(* Logix 5000 AddOnInstructionDefinition export EH_Cerabar_PMP23_IOL; software revision 38.00 *)

TYPE EH_CommAOI_Data :
STRUCT
   Device_Comm_Error : BOOL;
   CommSuccess : BOOL;
   CommFailed : BOOL;
   CommTimeOut : BOOL;
   StateDone : BOOL;
   NewState : BOOL;
   OldState : SINT;
   PortSize : SINT;
   DevicePort : SINT;
   MaxState : SINT;
   State : SINT;
   VendorID : INT;
   DeviceID : DINT;
   CyclicData : INT[16];
   AcyclicData : DINT[8];
   ReplayIndex : INT;
   AOI_Diagnostic : DINT;
   ConnectionStatus : DINT;
   OutputData : INT[16];
END_STRUCT
END_TYPE

ADD_ON_INSTRUCTION EH_Cerabar_PMP23_IOL   (* revision 1.0, vendor Endress+Hauser *)
// Cerabar PMP23 Rev 1 IO-Link
// Cerabar PMP23 Rev 2 IO-Link
// Cerabar PMP23 Rev 3 IO-Link
VAR_IN_OUT
   DataToSend : INT[10]; {required}
   CommAOIBusy : DINT; {required}
   ActiveComPort : DINT; {required}
   DeviceAOISendRequest : DINT; {required}
   CommError : INT; {required}
   DeviceData : EH_CommAOI_Data; {required}
END_VAR
VAR_INPUT
   iExecuteRisingEdge : BOOL; {visible}
   iGetZero : BOOL; {visible}
   iSetUnit : DINT; {visible}
END_VAR
VAR_OUTPUT
   qVendor_ID : DINT; {access Read Only, visible}
   qDevice_ID : DINT; {access Read Only, visible}
   qPressure : REAL; {visible}
   qCondensedStatus : USINT; {access Read Only, visible}
   qS_Out_1 : BOOL; {access Read Only, visible}
   qS_Out_2 : BOOL; {access Read Only, visible}
   qUnit : DINT; {access Read Only, visible}
   qAOI_Diagnostic : DINT; {access Read Only, visible}
END_VAR
VAR_IN_OUT
   qActual_Diagnostics_String : STRING; {required}
END_VAR
VAR_OUTPUT
   qActual_Diagnostics_Code : DINT; {access Read Only, visible}
END_VAR
VAR_IN_OUT
   qLast_Diagnostics_String : STRING; {required}
END_VAR
VAR_OUTPUT
   qLast_Diagnostics_Code : DINT; {access Read Only, visible}
   qCommunicationBusy : DINT; {visible}
   qCommError : DINT; {access Read Only, visible}
   qDeviceConnectionError : BOOL; {access None, visible}
END_VAR
VAR
   Calc_DID : DINT; {access None}
   Calc_VID : DINT; {access None}
   Calc_Data : DINT; {access None}
   Test : DINT; {access None}
   Pressure_DINT : DINT; {access None}
   Calc_Pressure : DINT; {access None}
   Calc_CondenStatus : DINT; {access None}
   CMD_Index : INT; {access None}
   CMD_Subindex : INT; {access None}
   CMD_ByteLength : INT; {access None}
   qDevice_ID_select : INT; {access None}
   Trigger : BOOL; {access None}
   CMD_Rd : BOOL; {access None}
   CMD_Wr : BOOL; {access None}
   Calc_Out : DINT; {access None}
   UnitSelection : REAL; {access None}
   InputByteLength : DINT;
   LocalChannel : BOOL; {access None}
   StateMin : DINT; {access None}
   StateMax : DINT; {access None}
   UseDeviceUnit : BOOL; {access None}
   ActiveAOI : BOOL; {access None}
   firstTimeDone : BOOL; {access None}
   AOI_Prio : BOOL; {access None}
   Calc_Connection_Status : DINT; {access None}
   DeviceID1 : DINT; {access None}
   DeviceID2 : DINT; {access None}
   DeviceID3 : DINT; {access None}
   qPressureTemp : REAL; {access None}
   FALSE : BOOL; {access None}
   TRUE : BOOL := 1; {access None}
END_VAR

ROUTINE Logic   (* structured text *)
// PMP23 Communication via AL1323
   // =======================================================================
   // Endress+Hauser Digital Solutions
   // ©Copyright (2024) All Rights Reserved
   // =======================================================================
   // Name:                EH_Cerabar_PMP23_IOL
   // Version:             1.0
   // Datum:               11.2025
   // Library:             01.01.00
   // Engineering:         Studio5000 V38.00.00
   // Author:              EH
   // =======================================================================
   
   
   qAOI_Diagnostic := DeviceData.AOI_Diagnostic;
   qCommunicationBusy := CommAOIBusy;
   DeviceID1 := 256;  //PMP 23 Rev 1
   DeviceID2 := 257;  //PMP 23 Rev 2
   DeviceID3 := 258;  //PMP 23 Rev 3
   StateMin := 0;
   DeviceData.MaxState := 6;
   
   if DeviceData.DevicePort = 0 or DeviceData.DeviceID < DeviceID1 or DeviceData.DeviceID > DeviceID3 or DeviceData.ConnectionStatus <> 1 then
   
   	qVendor_ID	:= 0;
   	qDevice_ID	:= 0;
   	qPressure	:= 0;
   	qS_Out_1	:= 0;
   	qS_Out_2	:= 0;
   	qCondensedStatus	:= 0;
   	qActual_Diagnostics_Code	:= 0;
   	qLast_Diagnostics_Code	:= 0;
   	qLast_Diagnostics_String	:= '';
   
   	if DeviceData.DevicePort = 0 then
   
   		qActual_Diagnostics_String	:= 'Device Port is Zero';
   		DeviceData.AOI_Diagnostic.1 := TRUE;
   
   	elsif DeviceData.ConnectionStatus <> 1 then
   
   		qActual_Diagnostics_String	:= 'No Device connected';
   		qDeviceConnectionError := TRUE;
   
   	elsif DeviceData.DeviceID < DeviceID1 or DeviceData.DeviceID > DeviceID3  then
   
   		qActual_Diagnostics_String	:= 'Wrong DeviceID';
   		DeviceData.AOI_Diagnostic.2 := TRUE;
   		qVendor_ID := DeviceData.VendorID;
   		qDevice_ID := DeviceData.DeviceID;
   
   	end_if;
   
   else
   
   	if qActual_Diagnostics_Code = 0 then
   
   		qActual_Diagnostics_String	:= '--------';
   
   	end_if;
   
   	if qLast_Diagnostics_Code = 0 then
   
   		qLast_Diagnostics_String	:= '--------';
   
   	end_if;
   
   	DeviceData.AOI_Diagnostic.1 := FALSE;
   	qDeviceConnectionError := FALSE;
   	DeviceData.AOI_Diagnostic.2  := FALSE;
   
   end_if;
   
   
   if not DeviceData.AOI_Diagnostic.0
   	and not qDeviceConnectionError
   	and not DeviceData.AOI_Diagnostic.2
   	and DeviceData.DevicePort > 0 or ActiveAOI and qDeviceConnectionError then
   
   	//*********************************
   	//Vendor ID
   	//*********************************
   
   	qVendor_ID := DeviceData.VendorID;
   
   	//*********************************
   	//Device ID
   	//*********************************
   
   	qDevice_ID := DeviceData.DeviceID;
   
   	if not UseDeviceUnit then
   
   		CASE iSetUnit OF
   
   			//*********************************
   			0: // Bar
   			//*********************************
   			UnitSelection := 10000.0;
   
   			//*********************************
   			1: // kPa
   			//*********************************
   			UnitSelection := 100.0;
   
   			//*********************************
   			2: // psi
   			//*********************************
   			UnitSelection := 1000.0;
   
   			//*********************************
   			3: // MPa
   			//*********************************
   			UnitSelection := 100000.0;
   
   		end_case;
   
   	end_if;
   
   	//*********************************
   	//Process Data Pressure
   	//*********************************
   	if DeviceData.DeviceID = DeviceID1 then
   
   		qDevice_ID_select := 1;
   
   	elsif DeviceData.DeviceID = DeviceID2 then
   
   		qDevice_ID_select := 2;
   
   	elsif DeviceData.DeviceID = DeviceID3 then
   
   		qDevice_ID_select := 3;
   
   	else
   
   		qDevice_ID_select := 0;
   
   	end_if;
   
   	case qDevice_ID_select of  // check for Different Version
   
   		//*********************************
   	    1: // PMP 23 Rev 1
   	    //*********************************
   
   		Calc_Pressure 	:= 0+((DeviceData.DevicePort-1)*InputByteLength);  // Value  95 + Protnumber x Datalength in Byte
   
   		Pressure_DINT :=  DeviceData.CyclicData[Calc_Pressure+1];
   		Pressure_DINT.8 :=  DeviceData.CyclicData[Calc_Pressure+1].8;
   		Pressure_DINT.9 :=  DeviceData.CyclicData[Calc_Pressure+1].9;
   		Pressure_DINT.10 :=  DeviceData.CyclicData[Calc_Pressure+1].10;
   		Pressure_DINT.11 :=  DeviceData.CyclicData[Calc_Pressure+1].11;
   		Pressure_DINT.12 :=  DeviceData.CyclicData[Calc_Pressure+1].12;
   		Pressure_DINT.13 :=  DeviceData.CyclicData[Calc_Pressure+1].13;
   		Pressure_DINT.14 :=  DeviceData.CyclicData[Calc_Pressure+1].14;
   		Pressure_DINT.15 :=  DeviceData.CyclicData[Calc_Pressure+1].15;
   		Pressure_DINT.16 :=  DeviceData.CyclicData[Calc_Pressure].0;
   		Pressure_DINT.17 :=  DeviceData.CyclicData[Calc_Pressure].1;
   		Pressure_DINT.18 :=  DeviceData.CyclicData[Calc_Pressure].2;
   		Pressure_DINT.19 :=  DeviceData.CyclicData[Calc_Pressure].3;
   		Pressure_DINT.20 :=  DeviceData.CyclicData[Calc_Pressure].4;
   		Pressure_DINT.21 :=  DeviceData.CyclicData[Calc_Pressure].5;
   		Pressure_DINT.22 :=  DeviceData.CyclicData[Calc_Pressure].5;
   		Pressure_DINT.23 :=  DeviceData.CyclicData[Calc_Pressure].5;
   		Pressure_DINT.24 :=  DeviceData.CyclicData[Calc_Pressure].5;
   		Pressure_DINT.25 :=  DeviceData.CyclicData[Calc_Pressure].5;
   		Pressure_DINT.26 :=  DeviceData.CyclicData[Calc_Pressure].5;
   		Pressure_DINT.27 :=  DeviceData.CyclicData[Calc_Pressure].5;
   		Pressure_DINT.28 :=  DeviceData.CyclicData[Calc_Pressure].5;
   		Pressure_DINT.29 :=  DeviceData.CyclicData[Calc_Pressure].5;
   		Pressure_DINT.30 :=  DeviceData.CyclicData[Calc_Pressure].5;
   		Pressure_DINT.31 :=  DeviceData.CyclicData[Calc_Pressure].5;
   
   
   		qPressure := Pressure_DINT;
   		qPressure := qPressure / UnitSelection;
   
   		//*********************************
   	    2: // PMP 23 Rev 2
   	    //*********************************
   
   		Calc_Pressure 	:= 0+((DeviceData.DevicePort-1)*InputByteLength);
   
   		Pressure_DINT :=  DeviceData.CyclicData[Calc_Pressure+1];
   		Pressure_DINT.8 :=  DeviceData.CyclicData[Calc_Pressure+1].8;
   		Pressure_DINT.9 :=  DeviceData.CyclicData[Calc_Pressure+1].9;
   		Pressure_DINT.10 :=  DeviceData.CyclicData[Calc_Pressure+1].10;
   		Pressure_DINT.11 :=  DeviceData.CyclicData[Calc_Pressure+1].11;
   		Pressure_DINT.12 :=  DeviceData.CyclicData[Calc_Pressure+1].12;
   		Pressure_DINT.13 :=  DeviceData.CyclicData[Calc_Pressure+1].13;
   		Pressure_DINT.14 :=  DeviceData.CyclicData[Calc_Pressure+1].14;
   		Pressure_DINT.15 :=  DeviceData.CyclicData[Calc_Pressure+1].15;
   		Pressure_DINT.16 :=  DeviceData.CyclicData[Calc_Pressure].0;
   		Pressure_DINT.17 :=  DeviceData.CyclicData[Calc_Pressure].1;
   		Pressure_DINT.18 :=  DeviceData.CyclicData[Calc_Pressure].2;
   		Pressure_DINT.19 :=  DeviceData.CyclicData[Calc_Pressure].3;
   		Pressure_DINT.20 :=  DeviceData.CyclicData[Calc_Pressure].4;
   		Pressure_DINT.21 :=  DeviceData.CyclicData[Calc_Pressure].5;
   		Pressure_DINT.22 :=  DeviceData.CyclicData[Calc_Pressure].6;
   		Pressure_DINT.23 :=  DeviceData.CyclicData[Calc_Pressure].7;
   		Pressure_DINT.24 :=  DeviceData.CyclicData[Calc_Pressure].8;
   		Pressure_DINT.25 :=  DeviceData.CyclicData[Calc_Pressure].9;
   		Pressure_DINT.26 :=  DeviceData.CyclicData[Calc_Pressure].10;
   		Pressure_DINT.27 :=  DeviceData.CyclicData[Calc_Pressure].11;
   		Pressure_DINT.28 :=  DeviceData.CyclicData[Calc_Pressure].12;
   		Pressure_DINT.29 :=  DeviceData.CyclicData[Calc_Pressure].13;
   		Pressure_DINT.30 :=  DeviceData.CyclicData[Calc_Pressure].13;
   		Pressure_DINT.31 :=  DeviceData.CyclicData[Calc_Pressure].13;
   
   		qPressure := Pressure_DINT;
   		qPressure := qPressure / UnitSelection;
   
   		//*********************************
   	    3: // PMP23 Rev 3
   	    //*********************************
   
   		Calc_Pressure 	:= 0+((DeviceData.DevicePort-1)*InputByteLength);
   		Calc_CondenStatus := 2+((DeviceData.DevicePort-1)*InputByteLength);
   
   		Pressure_DINT :=  DeviceData.CyclicData[Calc_Pressure+1];
   		Pressure_DINT.8 :=  DeviceData.CyclicData[Calc_Pressure+1].8;
   		Pressure_DINT.9 :=  DeviceData.CyclicData[Calc_Pressure+1].9;
   		Pressure_DINT.10 :=  DeviceData.CyclicData[Calc_Pressure+1].10;
   		Pressure_DINT.11 :=  DeviceData.CyclicData[Calc_Pressure+1].11;
   		Pressure_DINT.12 :=  DeviceData.CyclicData[Calc_Pressure+1].12;
   		Pressure_DINT.13 :=  DeviceData.CyclicData[Calc_Pressure+1].13;
   		Pressure_DINT.14 :=  DeviceData.CyclicData[Calc_Pressure+1].14;
   		Pressure_DINT.15 :=  DeviceData.CyclicData[Calc_Pressure+1].15;
   		Pressure_DINT.16 :=  DeviceData.CyclicData[Calc_Pressure].0;
   		Pressure_DINT.17 :=  DeviceData.CyclicData[Calc_Pressure].1;
   		Pressure_DINT.18 :=  DeviceData.CyclicData[Calc_Pressure].2;
   		Pressure_DINT.19 :=  DeviceData.CyclicData[Calc_Pressure].3;
   		Pressure_DINT.20 :=  DeviceData.CyclicData[Calc_Pressure].4;
   		Pressure_DINT.21 :=  DeviceData.CyclicData[Calc_Pressure].5;
   		Pressure_DINT.22 :=  DeviceData.CyclicData[Calc_Pressure].6;
   		Pressure_DINT.23 :=  DeviceData.CyclicData[Calc_Pressure].7;
   		Pressure_DINT.24 :=  DeviceData.CyclicData[Calc_Pressure].8;
   		Pressure_DINT.25 :=  DeviceData.CyclicData[Calc_Pressure].9;
   		Pressure_DINT.26 :=  DeviceData.CyclicData[Calc_Pressure].10;
   		Pressure_DINT.27 :=  DeviceData.CyclicData[Calc_Pressure].11;
   		Pressure_DINT.28 :=  DeviceData.CyclicData[Calc_Pressure].12;
   		Pressure_DINT.29 :=  DeviceData.CyclicData[Calc_Pressure].13;
   		Pressure_DINT.30 :=  DeviceData.CyclicData[Calc_Pressure].14;
   		Pressure_DINT.31 :=  DeviceData.CyclicData[Calc_Pressure].15;
   
   		COP(Pressure_DINT,qPressureTemp,1);
   
   		case qUnit of
   
   			//*********************************
   			0: // bar
   			//*********************************
   			qPressure := qPressureTemp / 100000;
   
   			//*********************************
   			1: // kPa
   			//*********************************
   			qPressure := qPressureTemp / 1000;
   
   			//*********************************
   			2: // psi
   			//*********************************
   			qPressure := qPressureTemp / 6895;
   
   			//*********************************
   			3: // MPA
   			//*********************************
   			qPressure := qPressureTemp / 1000000;
   
   			else // Base unit, Pa
   				qPressure := qPressureTemp;
   
   		end_case;
   
   	end_case;
   
   	//*********************************
   	// Process Parameter State IO1
   	//*********************************
   
   	if qDevice_ID = DeviceID1 then
   
   		qS_Out_1 :=  DeviceData.CyclicData[Calc_Pressure].6;
   		qS_Out_2 := 0;  // not supported
   
   	elsif qDevice_ID = DeviceID2 then
   
   		qS_Out_1 :=  DeviceData.CyclicData[Calc_Pressure].14;
   		qS_Out_2 := 0; // not supported
   
   	elsif qDevice_ID = DeviceID3 then
   
   		qS_Out_1 :=  DeviceData.CyclicData[Calc_CondenStatus].0;
   		qS_Out_2 :=  DeviceData.CyclicData[Calc_CondenStatus].1;
   
   	end_if;
   
   	//*********************************
   	// Process Parameter State IO1
   	//*********************************
   
   		if qDevice_ID = DeviceID3 then
   
   			qCondensedStatus.0 := DeviceData.CyclicData[Calc_CondenStatus].8;
   			qCondensedStatus.1 := DeviceData.CyclicData[Calc_CondenStatus].9;
   			qCondensedStatus.2 := DeviceData.CyclicData[Calc_CondenStatus].10;
   			qCondensedStatus.3 := DeviceData.CyclicData[Calc_CondenStatus].11;
   			qCondensedStatus.4 := DeviceData.CyclicData[Calc_CondenStatus].12;
   			qCondensedStatus.5 := DeviceData.CyclicData[Calc_CondenStatus].13;
   			qCondensedStatus.6 := DeviceData.CyclicData[Calc_CondenStatus].14;
   			qCondensedStatus.7 := DeviceData.CyclicData[Calc_CondenStatus].15;
   
   		end_if;
   
   	//*********************************
   	// Checking for CommBlockBusy
   	//*********************************
   
   
   	if iExecuteRisingEdge and DeviceData.State = 0 then
   
   		DeviceAOISendRequest.[DeviceData.DevicePort] := 1;
   
   	end_if;
   
   
   	if ActiveComPort = DeviceData.DevicePort then
   
   		AOI_Prio :=1;
   	else
   
   		AOI_Prio := 0;
   	end_if;
   
   
   	if CommAOIBusy = 1 and iExecuteRisingEdge and DeviceData.State = 0 and AOI_Prio then
   
   		ActiveAOI := 1;
   
   
   	end_if;
   
   
   	qCommunicationBusy := CommAOIBusy;
   	qAOI_Diagnostic := DeviceData.AOI_Diagnostic;
   
   	if  ActiveAOI and qDeviceConnectionError then
   
   		DeviceData.State := DeviceData.MaxState;
   
   	end_if;
   
   	//*********************************
   	// State machine
   	//*********************************
   
   
   	if ActiveAOI or DeviceData.State = DeviceData.MaxState then
   
   		case DeviceData.State of
   
   		    //*********************************
   		    0: // Idle
   		    //*********************************
   
   			    // Initializing reset to O for CMD Relevant Settings
   			    Trigger := 0;
   				CMD_Index := 0;
   				CMD_Subindex := 0;
   				CMD_Wr := 0;
   				CMD_Rd := 0;
   			    CMD_ByteLength := 0;
   
   				if DeviceData.DevicePort = ActiveComPort then // check if Device is Active to reset success
   						DeviceData.CommSuccess := 0;
   						DeviceData.CommTimeOut := 0;
   						DeviceData.NewState := 1;
   						DeviceData.StateDone := 0;
   				end_if;
   
   			    // Wait for trigger
   			    if iExecuteRisingEdge and ActiveComPort = DeviceData.DevicePort then
   
   					DeviceData.AOI_Diagnostic := 0;
   					DeviceData.State := DeviceData.State + 1;
   
   			    end_if;
   
   			//*********************************
   			1: // Set Unit
   			//*********************************
   
   				CMD_Index := 67;
   				CMD_Subindex := 0;
   				CMD_Wr := 1;								// Only Read or Write can be active = 1
   				CMD_Rd := 0;
   				CMD_ByteLength := 1;
   				DataToSend[6]:= 0;
   				DataToSend[7]:= 0;
   
   		        if iSetUnit >= 0 AND iSetUnit < 4 then		// Check if the value from outside is usable if not error set an go to next Step
   
   				   DataToSend[6].0 := iSetUnit.0;
   				   DataToSend[6].1 := iSetUnit.1;
   				   DataToSend[6].2 := iSetUnit.2;
   				   DataToSend[6].3 := iSetUnit.3;
   				   Trigger := 1;
   
   				   if DeviceData.NewState then
   
   						DeviceData.StateDone := 1;
   
   					end_if;
   
   				else
   
   		            DeviceData.AOI_Diagnostic.[DeviceData.State+7] := 1;
   					DeviceData.OldState := DeviceData.State;
   			        DeviceData.State := DeviceData.State + 1;
   					DeviceData.CommSuccess := 0;
   					DeviceData.AcyclicData[0] := 0;
   					DeviceData.NewState := 1;
   
   			    end_if;
   
   				if  DeviceData.CommSuccess and DeviceData.ReplayIndex = CMD_Index then
   
   					Trigger := 0;
   					DeviceData.OldState := DeviceData.State;
   			        DeviceData.State := DeviceData.State + 1;
   					DeviceData.CommSuccess := 0;
   					DeviceData.AcyclicData[0] := 0;
   					DeviceData.NewState := 1;
   
   				 elsif DeviceData.CommTimeOut then
   
   					DeviceData.AOI_Diagnostic.[DeviceData.State+7] := 1;
   					DeviceData.OldState := DeviceData.State;
   			        DeviceData.State := DeviceData.State + 1;
   					DeviceData.CommTimeOut := 0;
   					DeviceData.AcyclicData[0] := 0;
   					DeviceData.NewState := 1;
   
   			    end_if;
   
   		    //*********************************
   		    2: // Get Zero
   		    //*********************************
   
   		        CMD_Index := 69;
   		        CMD_Subindex := 0;
   		        CMD_Wr := 1;
   				CMD_Rd := 0;
   		        CMD_ByteLength := 1;
   				DataToSend[6]:= 0;
   				DataToSend[7]:= 0;
   
   				if DeviceData.NewState then
   
   					DeviceData.StateDone := 1;
   
   				end_if;
   
   				if iGetZero then
   
   					DataToSend[6].0 := 1;
   				else
   
   					DataToSend[6].0 := 0;
   				end_if;
   
   				Trigger := 1;
   
   				if  DeviceData.CommSuccess and DeviceData.ReplayIndex = CMD_Index then
   
   					Trigger := 0;
   					DeviceData.OldState := DeviceData.State;
   			        DeviceData.State := DeviceData.State + 1;
   					DeviceData.CommSuccess := 0;
   					DeviceData.AcyclicData[0] := 0;
   					DeviceData.NewState := 1;
   
   				 elsif DeviceData.CommTimeOut then
   
   					DeviceData.AOI_Diagnostic.[DeviceData.State+7] := 1;
   					DeviceData.OldState := DeviceData.State;
   			        DeviceData.State := DeviceData.State + 1;
   					DeviceData.CommTimeOut := 0;
   					DeviceData.AcyclicData[0] := 0;
   					DeviceData.NewState := 1;
   
   			    end_if;
   
   			//*********************************
   		    3: // Read Unit Set from Device
   		    //*********************************
   
   				CMD_Index := 67;
   		        CMD_Subindex := 0;
   		        CMD_Wr := 0;
   				CMD_Rd := 1;
   		        CMD_ByteLength := 1;
   				DataToSend[6]:= 0;
   				DataToSend[7]:= 0;
   				Trigger := 1;
   
   				if DeviceData.NewState then
   
   					DeviceData.StateDone := 1;
   
   				end_if;
   
   				if  DeviceData.CommSuccess and DeviceData.ReplayIndex = CMD_Index then
   
   					qUnit := DeviceData.AcyclicData[0];
   					UseDeviceUnit := 1;
   
   					CASE qUnit OF
   
   						//*********************************
   						0: // Bar
   						//*********************************
   						UnitSelection := 10000.0;
   
   						//*********************************
   						1: // kPa
   						//*********************************
   						UnitSelection := 100.0;
   
   						//*********************************
   						2: // psi
   						//*********************************
   						UnitSelection := 1000.0;
   
   						//*********************************
   						3: // MPa
   						//*********************************
   						UnitSelection := 100000.0;
   
   					end_case;
   
   					Trigger := 0;
   					DeviceData.OldState := DeviceData.State;
   			        DeviceData.State := DeviceData.State + 1;
   					DeviceData.CommSuccess := 0;
   					DeviceData.AcyclicData[0] := 0;
   					DeviceData.NewState := 1;
   
   				 elsif DeviceData.CommTimeOut then
   
   					DeviceData.AOI_Diagnostic.[DeviceData.State+7] := 1;
   					DeviceData.OldState := DeviceData.State;
   			        DeviceData.State := DeviceData.State + 1;
   					DeviceData.CommTimeOut := 0;
   					DeviceData.AcyclicData[0] := 0;
   					DeviceData.NewState := 1;
   
   			    end_if;
   
   			//*********************************
   		    4: // Actual Diagnostic
   		    //*********************************
   
   		        CMD_Index := 260;
   		        CMD_Subindex := 0;
   		        CMD_Wr := 0;
   				CMD_Rd := 1;
   				CMD_ByteLength := 2;
   				Trigger := 1;
   
   				if DeviceData.NewState then
   
   					DeviceData.StateDone := 1;
   
   				end_if;
   
   				if  DeviceData.CommSuccess and DeviceData.ReplayIndex = CMD_Index then
   
   					qActual_Diagnostics_Code	:= DeviceData.AcyclicData[0];
   
   					case qActual_Diagnostics_Code of
   
   
   				        16#3030_3030:
   				            qActual_Diagnostics_String := 'System ok';
   				        16#0000_0001:
   				            qActual_Diagnostics_String := 'no communication';
   				        16#5331_3430:
   				            qActual_Diagnostics_String := 'S140 Sensor signal outside of permitted ranges';
   				        16#4632_3730:
   				            qActual_Diagnostics_String := 'F270 Overpressure/lowpressure , Defect in electronics';
   				        16#4334_3331:
   				            qActual_Diagnostics_String := 'C431 Invalid position adjustment (current output)';
   				        16#4334_3332:
   				            qActual_Diagnostics_String := 'C432 Invalid position adjustment (switching output)';
   				        16#4634_3337:
   				            qActual_Diagnostics_String := 'F437 Incompatible configuration';
   				        16#4334_3639:
   				            qActual_Diagnostics_String := 'C469 Switch points output violated';
   				        16#4334_3835:
   				            qActual_Diagnostics_String := 'C485 Simulation active';
   				        16#5335_3130:
   				            qActual_Diagnostics_String := 'S510 Turn down violated';
   				        16#5338_3033:
   				            qActual_Diagnostics_String := 'S803 Current output not connected';
   				        16#4638_3034:
   				            qActual_Diagnostics_String := 'F804 Overload at switch otput';
   				        16#5339_3731:
   				            qActual_Diagnostics_String := 'S971 Measured value is outside sensor range';
   						else
   							qActual_Diagnostics_String := 'Error Code unknown';
   
   			 		end_case;
   
   					Trigger := 0;
   					DeviceData.OldState := DeviceData.State;
   			        DeviceData.State := DeviceData.State + 1;
   					DeviceData.CommSuccess := 0;
   					DeviceData.AcyclicData[0] := 0;
   					DeviceData.NewState := 1;
   
   				elsif DeviceData.CommTimeOut then
   
   					DeviceData.AOI_Diagnostic.[DeviceData.State+7] := 1;
   					Trigger := 0;
   					DeviceData.OldState := DeviceData.State;
   			        DeviceData.State := DeviceData.State + 1;
   					DeviceData.CommTimeOut := 0;
   					DeviceData.AcyclicData[0] := 0;
   					DeviceData.NewState := 1;
   
   			    end_if;
   
   			//*********************************
   		    5: // Last Diagnostic
   		    //*********************************
   
   		        CMD_Index := 261;
   				CMD_Subindex := 0;
   		        CMD_Wr := 0;
   				CMD_Rd := 1;
   				CMD_ByteLength := 2;
   		        Trigger := 1;
   
   				if DeviceData.NewState then
   
   					DeviceData.StateDone := 1;
   
   				end_if;
   
   				if  DeviceData.CommSuccess and DeviceData.ReplayIndex = CMD_Index then
   
   					qLast_Diagnostics_Code := DeviceData.AcyclicData[0];
   
   					case qLast_Diagnostics_Code of
   
   				        16#3030_3030:
   							qLast_Diagnostics_String := 'System ok';
   			        	16#0000_0001:
   							qLast_Diagnostics_String := 'no communication';
   				        16#5331_3430:
   							qLast_Diagnostics_String := 'S140 Sensor signal outside of permitted ranges';
   			        	16#4632_3730:
   							qLast_Diagnostics_String := 'F270 Overpressure/lowpressure , Defect in electronics';
   				        16#4334_3331:
   							qLast_Diagnostics_String := 'C431 Invalid position adjustment (current output)';
   				        16#4334_3332:
   							qLast_Diagnostics_String := 'C432 Invalid position adjustment (switching output)';
   			        	16#4634_3337:
   							qLast_Diagnostics_String := 'F437 Incompatible configuration';
   				        16#4334_3639:
   							qLast_Diagnostics_String := 'C469 Switch points output violated';
   			        	16#4334_3835:
   							qLast_Diagnostics_String := 'C485 Simulation active';
   				        16#5335_3130:
   							qLast_Diagnostics_String := 'S510 Turn down violated';
   			        	16#5338_3033:
   							qLast_Diagnostics_String := 'S803 Current loop, Current output not connected';
   			        	16#4638_3034:
   							qLast_Diagnostics_String := 'F804 Overload at switch otput';
   			        	16#5339_3731:
   							qLast_Diagnostics_String := 'S971 Measured value is outside sensor range';
   						else
   							qLast_Diagnostics_String := 'Error Code unknown';
   
   			 		end_case;
   
   					Trigger := 0;
   					DeviceData.OldState := DeviceData.State;
   			        DeviceData.State := DeviceData.State + 1;
   					DeviceData.CommSuccess := 0;
   					DeviceData.AcyclicData[0] := 0;
   					DeviceData.NewState := 1;
   
   				elsif DeviceData.CommTimeOut then
   
   					DeviceData.AOI_Diagnostic.[DeviceData.State+7] := 1;
   					Trigger := 0;
   					DeviceData.OldState := DeviceData.State;
   			        DeviceData.State := DeviceData.State + 1;
   					DeviceData.CommTimeOut := 0;
   					DeviceData.AcyclicData[0] := 0;
   					DeviceData.NewState := 1;
   
   			    end_if;
   
   			//*********************************
   		    6: // Trigger guard
   		    //*********************************
   
   				if not firstTimeDone then
   
   					CommAOIBusy := 0;
   					firstTimeDone := 1;
   					DeviceAOISendRequest.[DeviceData.DevicePort] := 0;
   					ActiveComPort := 0;
   					ActiveAOI := 0;
   					DataToSend[0] := 0;
   					DataToSend[1] := 0;
   					DataToSend[2] := 0;
   					DataToSend[3] := 0;
   					DataToSend[4] := 0;
   					DataToSend[5] := 0;
   					DataToSend[6] := 0;
   					DataToSend[7] := 0;
   					DataToSend[8] := 0;
   					DataToSend[9] := 0;
   					DeviceData.StateDone := 0;
   
   				end_if;
   
   				if DeviceData.State = DeviceData.MaxState AND NOT iExecuteRisingEdge then
   
   					DeviceData.State := 0;
   					DeviceData.OldState := DeviceData.State;
   					firstTimeDone := 0;
   
   				end_if;
   
   		end_case;
   	end_if;
   
   
   	//*************************
   	// Write Commands to the Master and the Device
   	//*************************
   	if DeviceData.State > StateMin and DeviceData.State < DeviceData.MaxState then
   
   		DataToSend[2] :=  DeviceData.DevicePort;
   		DataToSend[3] := CMD_Index;
   		DataToSend[4] := CMD_Subindex;
   		DataToSend[5].0 := CMD_Rd;
   		DataToSend[5].1 := CMD_Wr;
   		DataToSend[5].8 := CMD_ByteLength.0;
   		DataToSend[5].9 := CMD_ByteLength.1;
   		DataToSend[5].10 := CMD_ByteLength.2;
   		DataToSend[5].11 := CMD_ByteLength.3;
   		DataToSend[5].12 := CMD_ByteLength.4;
   		DataToSend[5].13 := CMD_ByteLength.5;
   		DataToSend[5].14 := CMD_ByteLength.6;
   		DataToSend[5].15 := CMD_ByteLength.7;
   
   		DataToSend[5].7 := Trigger;
   
   		qCommError	:= CommError;
   
   	end_if;
   
   end_if;
END_ROUTINE
END_ADD_ON_INSTRUCTION
